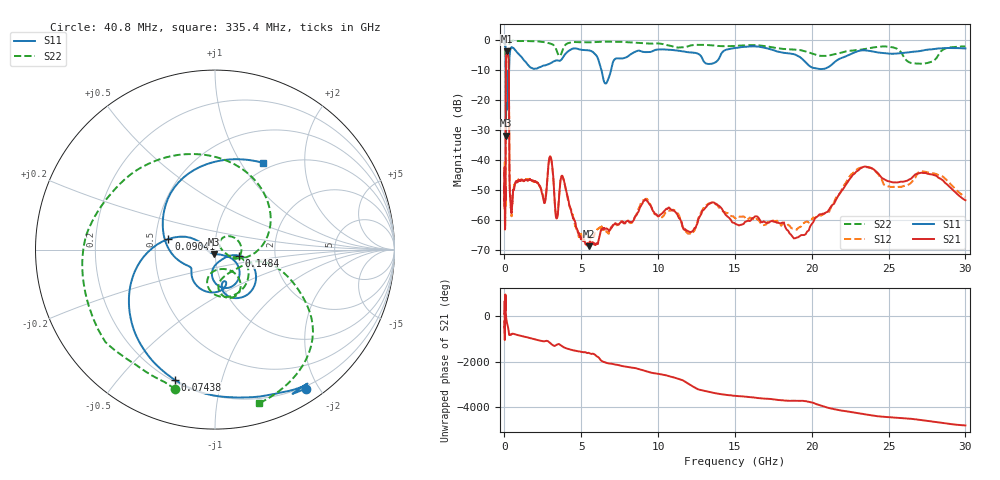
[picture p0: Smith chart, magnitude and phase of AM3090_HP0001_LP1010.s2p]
! Date/Time: Thu, Feb 28, 2019 1:54 PM
! Network Analyzer: Agilent Technologies E8364B Rev: A.07.50.67
! Sweep from 0.010 to 30.000 GHz, 1601 Points, Sweep Type: LOG
! Power Supply: 5.023 V, 0.002 A
# Hz S DB R 50
!freq MagS11 AngS11 MagS21 AngS21 MagS12 AngS12 MagS22 AngS22
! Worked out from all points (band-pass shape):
!   1601 points, 10 MHz to 30 GHz, reference 50 ohm
!   highest |S21| = -3.75 dB at 150.6 MHz (marker M1); lowest = -68.9 dB at 5.501 GHz (marker M2)
!   |S21| within 3 dB of the highest: 100.4 MHz to 270.3 MHz (170 MHz wide, 91.7 % of centre)
!   lowest |S11| = -32.0 dB at 98.93 MHz (marker M3), VSWR 1.05, Z = 49.5 - j2.47 ohm
!   |S11| at or under -10 dB: 89.6 MHz to 298.4 MHz (208.8 MHz wide, 108 % of centre); 6.309 GHz to 6.936 GHz (626.9 MHz wide, 9.47 % of centre)
!   |S22| runs from -29.9 to -0.2 dB; largest |S21 - S12| = 0.013
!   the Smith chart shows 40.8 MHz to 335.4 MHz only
!   S11 on the Smith chart (normalised r, x): 40.8 MHz: 0.17, -1.84; 74.38 MHz: 0.21, -0.72; 90.41 MHz: 0.58, +0.07; 148.4 MHz: 1.31, -0.09; 335.4 MHz: 0.90, +1.26
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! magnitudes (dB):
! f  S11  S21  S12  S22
! 10 MHz  -0.3  -51.0  -40.7  -0.7
! 38.04 MHz  -0.5  -63.2  -60.6  -1.6
! 40.8 MHz  -0.7  -62.1  -60.8  -1.9
! 74.38 MHz  -2.4  -47.1  -46.1  -4.4
! 90.41 MHz  -11.5  -14.9  -14.9  -11.5
! 98.93 MHz  -32.0  -7.2  -7.2  -29.0
! 114.4 MHz  -13.2  -4.9  -4.9  -18.5
! 144.7 MHz  -20.3  -3.8  -3.7  -18.5
! 148.4 MHz  -17.1  -3.8  -3.7  -17.5
! 150.6 MHz  -15.6  -3.7  -3.7  -16.8
! 274.6 MHz  -15.1  -7.4  -7.4  -16.2
! 335.4 MHz  -5.2  -47.9  -48.3  -1.0
! 550.5 MHz  -2.7  -50.7  -51.4  -0.3
! 2.084 GHz  -9.6  -47.5  -47.6  -0.5
! 2.61 GHz  -8.5  -54.5  -53.3  -0.7
! 3.002 GHz  -7.7  -39.0  -39.0  -1.2
! 3.368 GHz  -6.8  -59.5  -59.6  -3.1
! 3.798 GHz  -5.9  -45.8  -45.8  -3.2
! 5.501 GHz  -3.5  -68.9  -65.5  -0.8
! 7.926 GHz  -5.8  -60.7  -60.8  -0.7
! 23.48 GHz  -3.5  -42.3  -42.4  -3.0
! 30 GHz  -2.8  -53.5  -52.4  -2.2
